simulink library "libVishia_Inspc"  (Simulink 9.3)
settings: Solver=ode3  StartTime=0.0  StopTime=1  FixedStep=0.02/16384  RelTol=1e-3
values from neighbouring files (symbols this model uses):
  Tinit = 0.001    [TestOrthOsc_init.m]    (also in Test_PIDctrl_init.m)
undefined symbols (not defined in the file or in its folder): connection, from, intmax, name, name1Refl, name2Refl, simple, type, variable
libraries: $bdroot x1

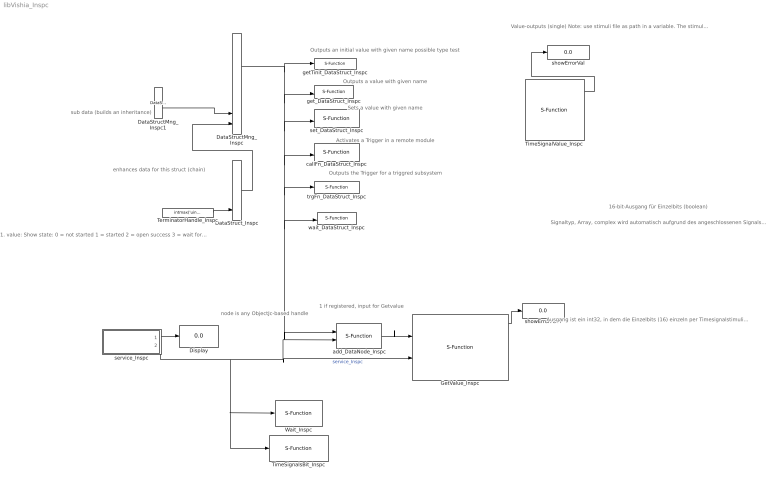
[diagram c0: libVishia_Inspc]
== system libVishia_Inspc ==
  note: 1 if registered, input for Getvalue
  note: node is any ObjectJc-based handle
  note: 1. value: Show state: 0 = not started 1 = started 2 = open success 3 = wait for receive 4 = execute received telg 5 = receive telg error, sleep 50 ms b =open error, wait for terminate d =should terminate f =terminated 2. value: count received telgs
  note: Outputs a value with given name
  note: Ausgang ist ein int32, in dem die Einzelbits (16) einzeln per Timesignalstimuli oder inspector belegt werden können. Parameter Name: Namen der Einzelbits. Werte in Timesignal-File: ==0 ist 0, !=0 setzt das Bit.
  note: Signaltyp, Array, complex wird automatisch aufgrund des angeschlossenen Signals erkannt. Es gibt teils Probleme mit back-probagation, wenn Simulink die Anzahl ArrayElemente nicht festlegen kann. Man muss dieses Problem lösen, indem die Leitung eindeutig bestimmt wird beispielsweise an den Ports. Hier kann man das Signal leider nicht bestimmen. . Sonderfunktion: Wenn Name mit * beginnt, dann muss der Eingang ein Pointer-Alias-Typ sein. Dann wird dessen Inhalt dargestellt.
  note: Value-outputs (single) Note: use stimuli file as path in a variable. The stimuli file can be a matlab script, with further initialization things. The stimuli-signals should be written as comment for matlab-script-language: %time:0.5: Signal=0.5, Signal2 = 0.7; Keyword is "%time:" * lines without this keyword are ignored - other matlab script statements. * More as one signal with the same time is possible, separated by comma. * Times need not be sorted, will be sorted internally. Parameter, configuration of signal names: ' Name in Reflection tree' for inspector access ** should be unique in the whole model. ** can contained in a String variable, especially for lib-modules (given as parameter) First output is error, 0: no error Last output is for data node.
  note: 16-bit-Ausgang für Einzelbits (boolean)
  note: Outputs an initial value with given name possible type test
  note: Sets a value with given name
  note: Activates a Trigger in a remote module
  note: Outputs the Trigger for a triggred subsystem
  note: sub data (builds an inheritance)
  note: enhances data for this struct (chain)
  DataStructMng_Inspc : S-Function  FunctionName=step_DataStructMng_Inspc_SfH  Parameters=dirGenSource typeData inputs inherit chain  SFunctionDeploymentMode=off  EnableBusSupport=off
  DataStructMng_Inspc1 : $bdroot/DataStructMng_Inspc  dirGenSource=''  typeData='TypeData'  inherit=off  chain=off  inputs="name;            //simple variable, type from connection"
  DataStruct_Inspc : S-Function  FunctionName=step_DataStruct_Inspc_SfH  Parameters=subn inputs  SFunctionDeploymentMode=off  EnableBusSupport=off
  Display : Display
  GetValue_Inspc : S-Function  FunctionName=get_GetValue_Inspc_SfH  Parameters=path1, path2, path3, path4, path5, path6, Tstep  SFunctionDeploymentMode=off  EnableBusSupport=off
  TerminatorHandle_Inspc : Constant  Value=intmax('uint32')  OutDataTypeStr=uint32  SampleTime=Tinit
  TimeSignalValue_Inspc : S-Function  Description=|  FunctionName=values_TimeSignals_Inspc_SfH  Parameters=Tstep filepath nameRefl nrofStimuli varDef  SFunctionDeploymentMode=off  EnableBusSupport=off
      | A combined stimuli and inspector function block.
      | Stimuli file path: file contains stimuli in form:
      |   %time:0: stimuli.namex = 5000.0, stimuli.namey = 50.0 -10; 
      | Name in reflection-tree: Name of this function block for stimuli and inspector access
      | name1..12: output type and name, base type is single always.
      | C2:namexy  A complex array of 2 elements
      | 6:namexy An array of 6 elements (max).
      | C:namexy  A 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
  TimeSignalsBit_Inspc : S-Function  Commented=on  FunctionName=TimeSignalsBit_Inspc_mex  Parameters=filepath nameRefl nrofStimuli n1 n2 n3 n4 n5 n6 n7 n8 n9 n10 n11 n12 n13 n14 n15 n16  SFunctionDeploymentMode=off  EnableBusSupport=off
  Wait_Inspc : S-Function  Commented=on  FunctionName=step_Wait_Inspc_SfH  Parameters=Tstep cyclesStart delay_ms  SFunctionDeploymentMode=off  EnableBusSupport=off
  add_DataNode_Inspc : S-Function  FunctionName=addObj_DataNode_Inspc_SfOp  Parameters=name1Refl name2Refl  SFunctionDeploymentMode=off  EnableBusSupport=off
  callFn_DataStruct_Inspc : S-Function  FunctionName=callFn_Access_DataStruct_Inspc_SfH  Parameters=name1 '' '' Tstep  SFunctionDeploymentMode=off  EnableBusSupport=off
  getTinit_DataStruct_Inspc : S-Function  FunctionName=getTinit_Access_DataStruct_Inspc_SfH  Parameters=typeName headerfile  SFunctionDeploymentMode=off  EnableBusSupport=off
  get_DataStruct_Inspc : S-Function  FunctionName=get_Access_DataStruct_Inspc_SfH  Parameters=name1 headerfile Tstep  SFunctionDeploymentMode=off  EnableBusSupport=off
  service_Inspc : Subsystem
  set_DataStruct_Inspc : S-Function  FunctionName=set_Access_DataStruct_Inspc_SfH  Parameters=typeName headerfile Tstep  SFunctionDeploymentMode=off  EnableBusSupport=off
  showErrorPath : Display
  showErrorVal : Display
  trgFn_DataStruct_Inspc : S-Function  FunctionName=trgFn_Access_DataStruct_Inspc_SfH  Parameters=name1 'F' name1 Tstep  SFunctionDeploymentMode=off  EnableBusSupport=off
  wait_DataStruct_Inspc : S-Function  FunctionName=wait_Access_DataStruct_Inspc_SfH  Parameters=usWait msTimeout name1 headerfile Tstep  SFunctionDeploymentMode=off  EnableBusSupport=off
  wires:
  service_Inspc/2(Out1) -> Wait_Inspc/1, TimeSignalsBit_Inspc/1, add_DataNode_Inspc/2, GetValue_Inspc/2  "service_Inspc"
  GetValue_Inspc/1 -> showErrorPath/1
  TimeSignalValue_Inspc/1 -> showErrorVal/1
  service_Inspc/1(Out2) -> Display/1
  add_DataNode_Inspc/1 -> GetValue_Inspc/1
  DataStructMng_Inspc/1 -> getTinit_DataStruct_Inspc/1, get_DataStruct_Inspc/2, callFn_DataStruct_Inspc/2, wait_DataStruct_Inspc/2, add_DataNode_Inspc/1, trgFn_DataStruct_Inspc/1, set_DataStruct_Inspc/2
  DataStruct_Inspc/1 -> DataStructMng_Inspc/9
  DataStructMng_Inspc1/2 -> DataStructMng_Inspc/8
  TerminatorHandle_Inspc/1 -> DataStruct_Inspc/5

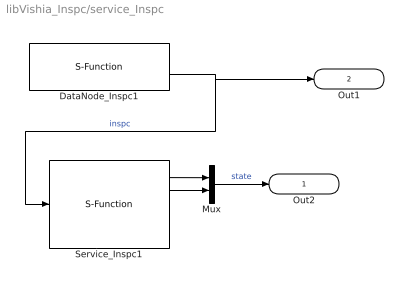
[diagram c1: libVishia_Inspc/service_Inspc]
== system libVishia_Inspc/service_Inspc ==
  DataNode_Inspc1 : S-Function  FunctionName=create_DataNode_Inspc_SfH  Parameters=50, Tstep  SFunctionDeploymentMode=off  EnableBusSupport=off
  Mux : Mux  Inputs=2
  Service_Inspc1 : S-Function  FunctionName=step_Service_Inspc_SfH  Parameters=Tstep, IpPort  SFunctionDeploymentMode=off  EnableBusSupport=off
  Out2 : Outport
  Out1 : Outport  Port=2  OutDataTypeStr=uint32  PortDimensions=1
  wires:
  DataNode_Inspc1/2 -> Service_Inspc1/1, Out1/1  "inspc"
  Mux/1 -> Out2/1  "state"
  Service_Inspc1/2 -> Mux/2
  Service_Inspc1/1 -> Mux/1
